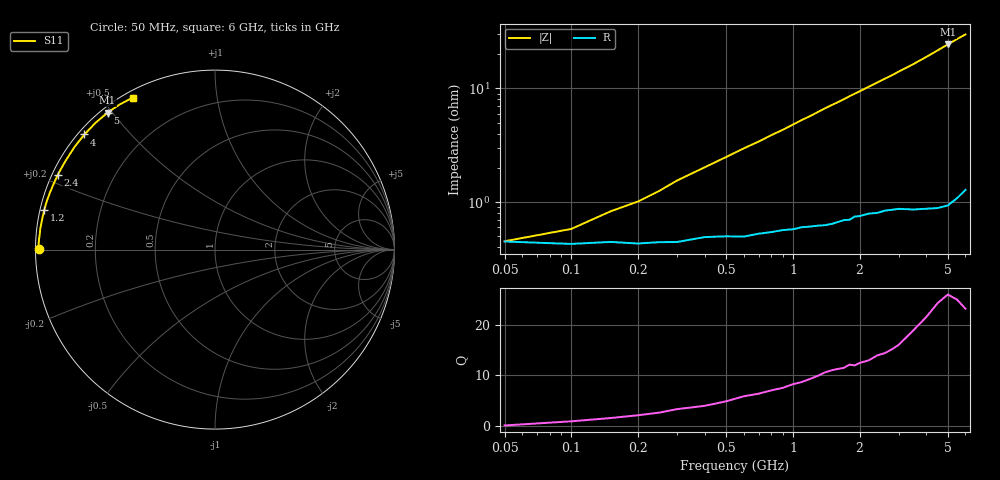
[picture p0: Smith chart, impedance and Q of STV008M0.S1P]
! SIEMENS Discrete & RF Semiconductors
! BA892
! Si PIN Diode in SCD-80
! IF = 8 mA
! S-Parameters:  September  1997
# GHz  S  MA  R  50
!  f  S11
! GHz  MAG  ANG
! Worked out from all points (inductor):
!   34 points, 50 MHz to 6 GHz, reference 50 ohm
!   read as one part to ground: L = 782 pH near 300 MHz
!   highest Q = 25 at 5 GHz (marker M1), where L = 774 pH
!   S11 on the Smith chart (normalised r, x): 50 MHz: 0.01, +0.00; 1.2 GHz: 0.01, +0.11; 2.4 GHz: 0.02, +0.22; 4 GHz: 0.02, +0.38; 5 GHz: 0.02, +0.49; 6 GHz: 0.03, +0.59
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0.05  0.9821 179.9
0.1  0.983 179.1
0.15  0.9823 178.4
0.2  0.9828 177.9
0.25  0.9824 177.3
0.3  0.9823 176.6
0.4  0.9805 175.5
0.6  0.9803 173.3
0.7  0.9792 172.3
0.8  0.9785 171.2
0.9  0.9777 170.2
1.1  0.9764 168.0
1.2  0.9762 167.0
1.4  0.9756 164.8
1.6  0.9741 162.8
1.7  0.9732 161.8
1.8  0.9731 160.7
1.9  0.9714 159.7
2.4  0.9698 154.7
2.6  0.9687 152.7
2.8  0.9684 150.8
3  0.9681 148.7
3.5  0.9693 143.8
4  0.9698 138.6
4.5  0.9705 133.3
5  0.9702 128.1
5.5  0.9671 123.1
6  0.9628 118.5
